{attribute 'qualified_only'}
VAR_GLOBAL CONSTANT
	//Disable drive
	DISABLE:USINT				:= 0;
	//Enable drive
	ENABLE:USINT				:= 1;
	//Clear start motion (enable drive
	CLEAR_START_MOTION:USINT 	:= 1;
	//Start motion
	START_MOTION:USINT 			:= 3;
	//Execute home move
	HOME:USINT 					:= 5;
	//Software stop (estop) at max deceleration
	SOFTWARE_STOP:USINT 		:= 8;
	//Stop motion at profile deceleration
	STOP_MOTION:USINT 			:= 17;
	//Declare current position home
	HOME_HERE:USINT 			:= 21;
	
END_VAR
